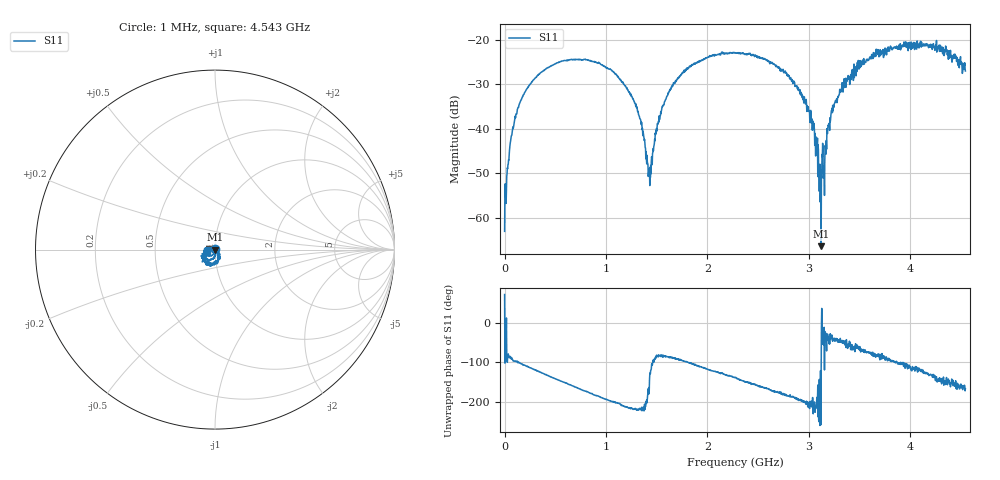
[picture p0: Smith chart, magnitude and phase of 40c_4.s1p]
# HZ S RI R 50
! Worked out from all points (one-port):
!   1515 points, 1 MHz to 4.543 GHz, reference 50 ohm
!   lowest |S11| = -66.4 dB at 3.121 GHz (marker M1), VSWR 1.00, Z = 50 - j0.0395 ohm
!   |S11| at or under -10 dB: start of sweep to end of sweep
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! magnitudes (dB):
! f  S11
! 1 MHz  -63.1
! 25 MHz  -50.1
! 61 MHz  -42.6
! 148 MHz  -34.3
! 319 MHz  -28.1
! 571 MHz  -24.7
! 919 MHz  -25.3
! 1.138 GHz  -28.7
! 1.318 GHz  -36.2
! 1.423 GHz  -49.6
! 1.546 GHz  -36.0
! 1.705 GHz  -28.7
! 2.002 GHz  -23.9
! 2.272 GHz  -22.8
! 2.575 GHz  -24.4
! 2.842 GHz  -29.8
! 3.034 GHz  -40.3
! 3.073 GHz  -42.7
! 3.103 GHz  -54.1
! 3.121 GHz  -66.4
! 3.133 GHz  -46.3
! 3.181 GHz  -40.8
! 3.238 GHz  -36.0
! 3.409 GHz  -28.9
! 3.655 GHz  -23.3
! 3.976 GHz  -21.1
! 4.291 GHz  -21.4
! 4.543 GHz  -27.0
